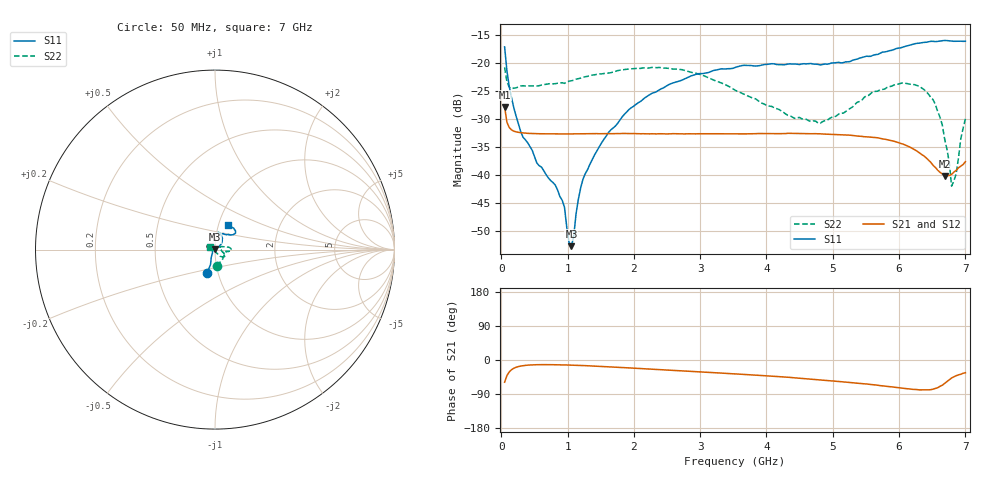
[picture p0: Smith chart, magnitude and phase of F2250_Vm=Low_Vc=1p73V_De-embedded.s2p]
! Integrated Device Technology
! Corporate Headquarters
! 6024 Silver Creek Valley Road
! San Jose, CA 95138  USA
! Phone:  1-408-284-8200
! Toll Free:  1-800-223-1366
! Webpage:  http://www.idt.com/
! Timing and RF Division
! 515 Groton Road, Suite 102
! Westford, MA 01886-6024
! Device:  F2250
! Description: Voltage Variable RF Attenuator
! Frequency:  50.0 -  6000.00 MHz
! Package:  3x3 mm Thin QFN Plastic Package: 16 pin
! Ports:  2 RF, 3 DC
!  Pin  1  = GND
!  Pin  2  = NC
!  Pin  3  = RF1  = Port 1
!  Pin  4  = NC
!  Pin  5  = GND
!  Pin  6  = GND
!  Pin  7  = GND
!  Pin  8  = GND
!  Pin  9  = NC
!  Pin 10  = RF2  = Port 2
!  Pin 11  = NC
!  Pin 12  = GND
!  Pin 13  = GND
!  Pin 14  = VCNTRL
!  Pin 15  = VDD
!  Pin 16  = VMODE
! Vcntrl:  1.730 Volts
! Vmode:  +0.000 Volts
! Vdd:  +3.30  Volts
! Current:  1.186 mA
! Data:  The device was measured on a the F2250 evaluation board which has
!  individual transmission lines to the RF pins.  Data was collected
!  using a calibrated network analyzer.  The evaluation board was
!  de-embedded using a TRL calibration technique.
!  The reference plane is the edge of the package pin.
! Misc:  SN 10
!  Action Tracker AT0258
! Date Measured:  2014-11-26
! Date:  2015-10-15  MJV
! Note:
!  Integrated Device Technology supplies this data as a sample of measured
!  data at the package pin for this product.  Your particular data for this
!  product may vary.
!  Data was taken at 25 degrees C.
!  Integrated Device Technology reserves the right to change this data at anytime.
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# GHz S dB R 50
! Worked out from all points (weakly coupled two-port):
!   201 points, 50 MHz to 7 GHz, reference 50 ohm
!   highest |S21| = -27.91 dB at 50 MHz (marker M1); lowest = -40.2 dB at 6.687 GHz (marker M2)
!   lowest |S11| = -52.8 dB at 1.058 GHz (marker M3), VSWR 1.00, Z = 49.9 + j0.213 ohm
!   |S11| at or under -10 dB: start of sweep to end of sweep
!   |S22| runs from -42.0 to -20.8 dB; largest |S21 - S12| = 9.9e-05
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0.05  -17.16 -108.1  -27.91 -58.6  -27.91 -58.5  -20.81 -83.3
0.1195  -24.20 -111.0  -31.56 -31.5  -31.59 -31.5  -24.36 -35.5
0.29325  -32.31 -126.1  -32.49 -16.0  -32.49 -16.0  -24.15 -15.0
0.91875  -44.59 157.7  -32.72 -12.9  -32.74 -12.9  -23.57 -9.1
0.9535  -45.83 171.0  -32.73 -13.0  -32.74 -13.0  -23.68 -8.6
1.023  -52.18 139.4  -32.71 -13.4  -32.71 -13.4  -23.29 -7.9
1.05775  -52.78 111.7  -32.71 -13.5  -32.71 -13.5  -23.22 -7.7
1.162  -44.42 49.5  -32.69 -14.1  -32.70 -14.1  -22.84 -8.6
1.2315  -40.81 40.0  -32.70 -14.6  -32.68 -14.6  -22.61 -9.0
1.6485  -32.03 40.4  -32.69 -18.1  -32.67 -18.1  -21.78 -5.9
2.37825  -24.88 46.6  -32.69 -25.1  -32.67 -25.2  -20.84 0.2
3.525  -20.85 72.1  -32.71 -36.6  -32.71 -36.6  -24.89 15.2
4.7065  -20.22 72.1  -32.67 -50.9  -32.67 -50.9  -30.39 15.7
5.85325  -17.85 40.2  -33.84 -70.3  -33.84 -70.4  -24.27 -30.8
6.40925  -16.33 41.6  -37.00 -79.0  -37.02 -79.0  -25.15 -46.2
6.54825  -16.21 45.0  -38.72 -75.0  -38.72 -75.0  -27.49 -53.5
6.68725  -16.01 48.6  -40.24 -61.8  -40.25 -61.6  -33.63 -64.3
6.75675  -16.08 51.0  -40.14 -52.5  -40.15 -52.5  -37.78 -81.7
6.7915  -16.12 52.1  -39.95 -47.5  -39.93 -47.4  -42.05 -109.4
6.861  -16.15 54.9  -39.23 -41.5  -39.19 -41.6  -39.81 -169.5
6.9305  -16.14 59.1  -38.48 -37.7  -38.47 -37.6  -33.59 159.6
7  -16.15 63.1  -37.67 -33.6  -37.65 -33.5  -30.02 149.1
